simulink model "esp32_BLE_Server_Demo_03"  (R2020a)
settings: Solver=FixedStepDiscrete  StartTime=0.0  StopTime=10.0  RelTol=1e-3  EnableMultiTasking=on
undefined symbols (not defined in the file): BLE_demo, CR, demo, Demo_03, ESP, esp32, esp32_BLE_Server_Demo_03_esp32_build_system, float, IDF, In1, In2, IP, Out1, Out2, Param1, r, Server, SPP_BLE, targets, TCP, Trunk, uint32_t, waijung2
libraries: simulink x4, esp32_ble_lib x2, waijung2_utilities_lib x1, esp32_device_config_lib x1

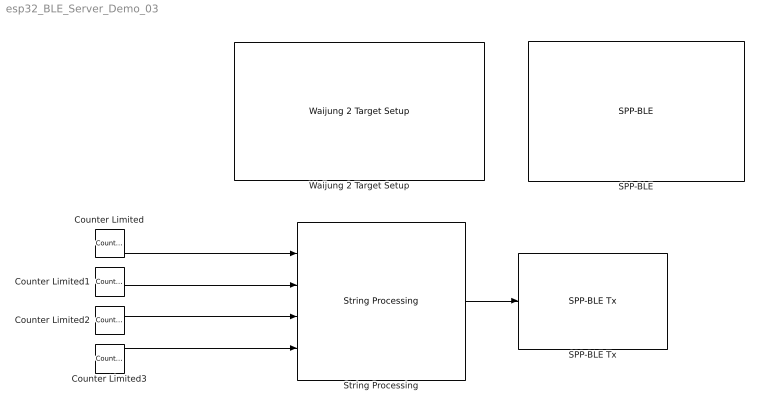
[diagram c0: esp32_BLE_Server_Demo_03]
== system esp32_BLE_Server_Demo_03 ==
  Counter Limited : simulink/Sources/Counter Limited  uplimit=100  tsamp=1
  Counter Limited1 : simulink/Sources/Counter Limited  uplimit=10  tsamp=-1
  Counter Limited2 : simulink/Sources/Counter Limited  uplimit=5  tsamp=-1
  Counter Limited3 : simulink/Sources/Counter Limited  uplimit=20  tsamp=-1
  SPP-BLE : esp32_ble_lib/SPP-BLE  conf=Setup  spp=Server  ssid=BLE Server Demo 2  uartmodule=0  baudrate=115200  databits=8  parity=None  stopbit=1  txpin=32  rxpin=33  advanceoptions=on  rxbuffersize=256  txbuffersize=256  porttype_double=0  porttype_single=0  porttype_int8=0  porttype_uint8=0  porttype_int16=0  porttype_uint16=0  porttype_int32=0  porttype_uint32=2  asciiformat='Value=%1.2f'  tx_asciiterminator="CR (0x0D - \"\\r\")"  rx_asciiterminator="CR (0x0D - \"\\r\")"  buffersize=128  storagename=1  portpinstr=0  sampletime=-1  enablecustomportlabel=off  cinputportlabel=In1,In2  coutputportlabel=Out1,Out2  blockid=SPPBLE  inputporttype=[]  inputportwidth=[]  inputportlabel={}  outputporttype=[]  outputportwidth=[[]]  outputportlabel={}  compat=0  optionstring="[\"0\",\"115200\",\"Server\",\"BLE Server Demo 2\",\"256\",\"256\",\"Value=%1.2f\",\"\",\"\",\"UART_DATA_8_BITS\",\"UART_PARITY_DISABLE\",\"UART_STOP_BITS_1\",\"128\"]"  optionstring2="[\"float\"]"  MsgBufferSize=16
  SPP-BLE Tx : esp32_ble_lib/SPP-BLE Tx  conf=Tx  spp=Server  ssid=BLE SPP Server  uartmodule=0  databits=8  parity=None  stopbit=1  txpin=32  rxpin=33  advanceoptions=on  rxbuffersize=256  txbuffersize=256  porttype_double=0  porttype_single=0  porttype_int8=0  porttype_uint8=0  porttype_int16=0  porttype_uint16=0  porttype_int32=0  porttype_uint32=2  asciiformat='Joystick_Values=%s'  baudrate=Consistent  tx_asciiterminator="CR (0x0D - \"\\r\")"  rx_asciiterminator="CR (0x0D - \"\\r\")"  buffersize=128  storagename=1  portpinstr=0  sampletime=-1  enablecustomportlabel=off  cinputportlabel=In1,In2  coutputportlabel=Out1,Out2  blockid=SPPBLETx  inputporttype=[3]  inputportwidth=64  inputportlabel={'string'}  outputporttype=[]  outputportwidth=[[]]  outputportlabel={}  compat=0  optionstring="[\"0\",\"Consistent\",\"Server\",\"BLE SPP Server\",\"256\",\"256\",\"Joystick_Values=%s\",\"0x0D\",\"1\",\"UART_DATA_8_BITS\",\"UART_PARITY_DISABLE\",\"UART_STOP_BITS_1\",\"128\"]"  optionstring2="[\"char *\"]"  txdatatype='string'  MsgBufferSize=64
  String Processing : waijung2_utilities_lib/String Processing  conf=processing  stringfunction=sprintf  stringformat='%u,%u,%u,%u'  begindelimiter=''  enddelimiter=''  buffersize=64  enablestatus=off  use_pointer=off  pointer_list="\"\""  string_pointer=off  portpinstr=0  sampletime=-1  blockid=StringProcessing  inputporttype=[-1 -1 -1 -1]  inputportwidth=[1 1 1 1]  inputportlabel={'%u','%u','%u','%u'}  outputporttype=[3]  outputportwidth=[64]  outputportlabel={'Output'}  compat=0  optionstring="[\"Param1\",\"Param1\"]"  datatypestring="[\"uint32_t\",\"uint32_t\",\"uint32_t\",\"uint32_t\"]"
  Waijung 2 Target Setup : esp32_device_config_lib/Waijung 2 Target Setup  waijungversion=22.12a  toolchain=ESP-IDF  os=FreeRTOS  sampletime=-1  simulink_managebuildsystem=on  projectpath=E:\Trunk\waijung2\targets\esp32\demo\BLE_demo\SPP_BLE\Demo_03\Server\esp32_BLE_Server_Demo_03_esp32_build_system  espidfpath=C:\msys32\home\skris\esp\esp-idf  buildoptions=Deploy to hardware  blockid=Waijung2TargetSetup  target=ESP32  defaultstacksize=4086  basepriority=0  highestpriority=10  generate_baserate_task=on  tickrate=1000  esp32target=ESP32  esp32targetdef=esp32  esp32flashsize=4MB  esp32comport=COM3  esp32baudrate=115200  esp32advancedconfig=on  esp32partitiontable=Use default waijung2 partition table  esp32partitionpath=Browse the partition table  partitionname=partitions.csv  editpartition=on  custompartitiondata={'nvs','data','nvs','','0x6000','';'phy_init','data','phy','','0x1000','';'factory','app','factory','','1M',''}  reqblocks=default  esp32custompartition={'nvs','data','nvs','','0x6000','';'phy_init','data','phy','','0x1000','';'factory','app','factory','','1M',''}  cominterface=TCP/IP  uart_module=0  baudrate=115200  tx_pin=0  rx_pin=0  com_port=9  wifimode=WIFI AP  wifissid=esp32ssid  wifipassword=password  deviceip=192.168.1.10  targetgateway=192.168.1.1  targetnetmask=255.255.255.0  manualdns=on  targetdnsip=8.8.8.8  targetipport=256  targetipdef=0  targetmaskdef=0  targetgatewaydef=0  targetdnsipdef=0  hosttimeout=10  hostverbose=off
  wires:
  String Processing/1 -> SPP-BLE Tx/1
  Counter Limited/1 -> String Processing/1
  Counter Limited1/1 -> String Processing/2
  Counter Limited2/1 -> String Processing/3
  Counter Limited3/1 -> String Processing/4
